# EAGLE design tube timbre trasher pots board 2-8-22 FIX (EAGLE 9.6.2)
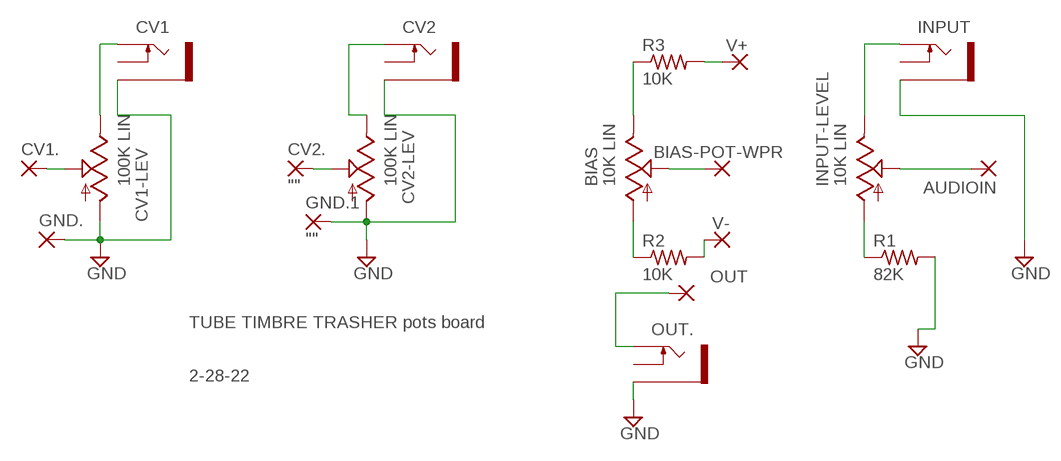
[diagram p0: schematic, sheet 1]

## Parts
AUDIOIN  WIREPAD3,17/1,3  [3,17/1,3]
BIAS  10K LIN  9MM_SNAP-IN_POT_  [9MM_SNAP-IN_POT]
BIAS-POT-WPR  WIREPAD3,17/1,3  [3,17/1,3]
CV1  THONKICONNNEW  [WQP-PJ301M-12_JACK]
CV1-LEV  100K LIN  9MM_SNAP-IN_POT_  [9MM_SNAP-IN_POT]
CV1.  WIREPAD3,17/1,3  [3,17/1,3]
CV2  THONKICONNNEW  [WQP-PJ301M-12_JACK]
CV2-LEV  100K LIN  9MM_SNAP-IN_POT_  [9MM_SNAP-IN_POT]
CV2.  ""  WIREPAD3,17/1,3  [3,17/1,3]
GND.  WIREPAD3,17/1,3  [3,17/1,3]
GND.1  ""  WIREPAD3,17/1,3  [3,17/1,3]
INPUT  THONKICONNNEW  [WQP-PJ301M-12_JACK]
INPUT-LEVEL  10K LIN  9MM_SNAP-IN_POT_  [9MM_SNAP-IN_POT]
OUT  WIREPAD3,17/1,3  [3,17/1,3]
OUT.  THONKICONNNEW  [WQP-PJ301M-12_JACK]
R1  82K  R-US_0207/10  [0207/10]
R2  10K  R-US_0207/10  [0207/10]
R3  10K  R-US_0207/10  [0207/10]
V+  WIREPAD3,17/1,3  [3,17/1,3]
V-  WIREPAD3,17/1,3  [3,17/1,3]

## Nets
GND: CV1-LEV.1(A) CV1.P$3_SLEEVE(SLEEVE) CV2-LEV.1(A) CV2.P$3_SLEEVE(SLEEVE) GND.1.1(P) GND..1(P) INPUT.P$3_SLEEVE(SLEEVE) OUT..P$3_SLEEVE(SLEEVE) R1.2
N$1: INPUT-LEVEL.3(E) INPUT.P$1_TIP(TIP)
N$2: AUDIOIN.1(P) INPUT-LEVEL.2(S)
N$3: BIAS.3(E) R3.1
N$4: OUT.1(P) OUT..P$1_TIP(TIP)
N$5: CV1-LEV.3(E) CV1.P$1_TIP(TIP)
N$6: CV2-LEV.3(E) CV2.P$1_TIP(TIP)
N$7: CV1-LEV.2(S) CV1..1(P)
N$8: CV2-LEV.2(S) CV2..1(P)
N$9: BIAS.1(A) R2.1
N$10: BIAS-POT-WPR.1(P) BIAS.2(S)
N$12: INPUT-LEVEL.1(A) R1.1
N$13: R3.2 V+.1(P)
N$14: R2.2 V-.1(P)
Unconnected: CV1.P$2_SWITCH(SWITCH) CV2.P$2_SWITCH(SWITCH) INPUT.P$2_SWITCH(SWITCH) OUT..P$2_SWITCH(SWITCH)

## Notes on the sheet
- TUBE TIMBRE TRASHER pots board
- 2-28-22

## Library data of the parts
AUDIOIN BIAS-POT-WPR CV1. CV2. GND. GND.1 OUT V+ V- = wirepad:WIREPAD: Wire PAD connect wire on PCB
BIAS CV1-LEV CV2-LEV INPUT-LEVEL = MusicThingModular:9MM_SNAP-IN_POT: 9mm vertical snap-in pot, Alpha / Panasonic style
CV1 CV2 INPUT OUT. = MusicThingModular-CL:THONKICONN: 3.5mm socket for Eurorack modular synths
R1-R3 = adafruit:R-US_: RESISTOR, American symbol

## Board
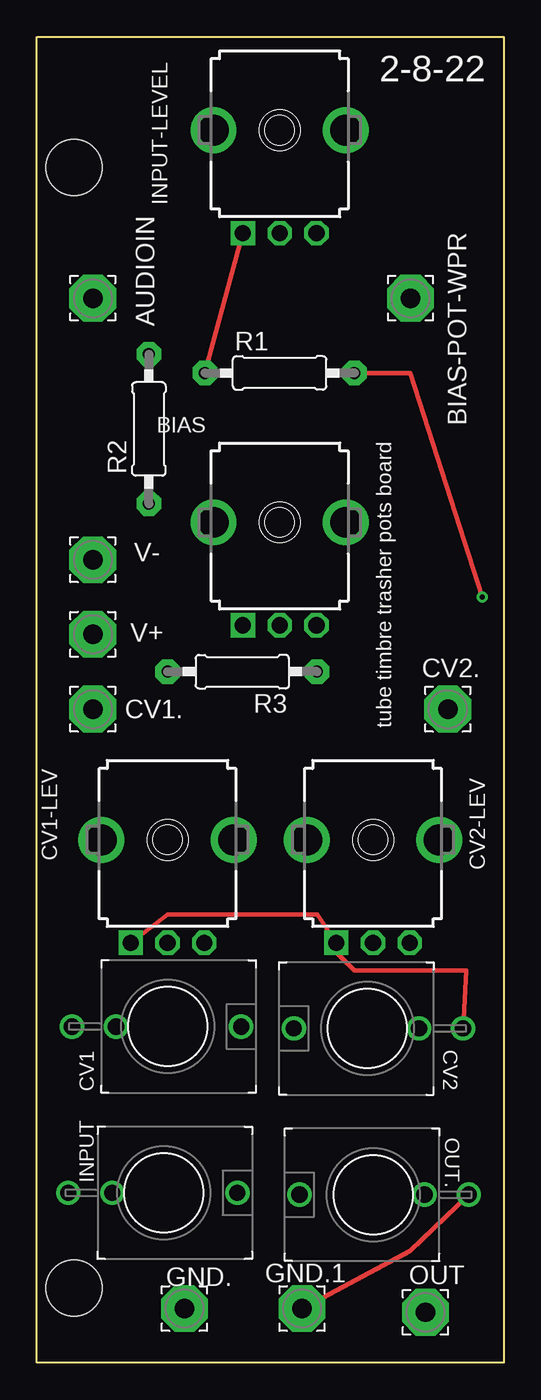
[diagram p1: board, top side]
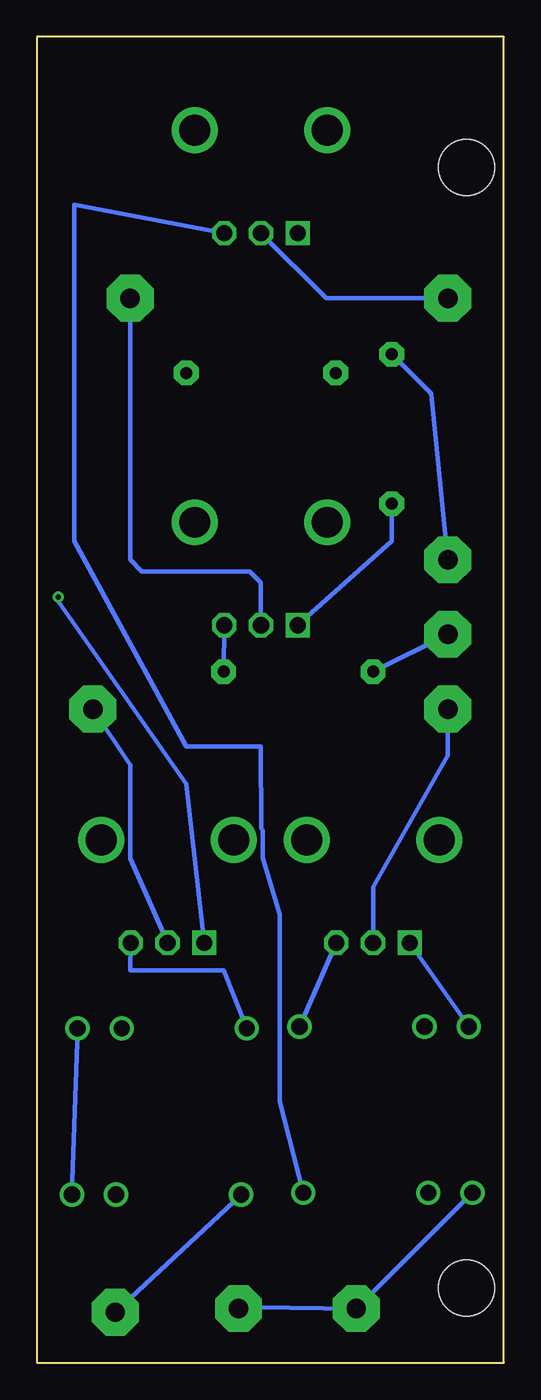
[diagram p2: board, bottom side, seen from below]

Size 31.75 x 90.17 mm. Coordinates in mm from the lower left corner, seen from the top.
Outline: 0,0 0,90.17 31.75,90.17 31.75,0 0,0
Copper layers (1*16): Top 0.035mm / dielectric 1.5mm / Bottom 0.035mm
Design rules "default": minimum track width 6mil, minimum drill 0.35mm, track to track 6mil, track to pad 6mil, pad to pad 6mil, via to via 6mil, smd to smd 6mil, copper to edge 40mil, drill to drill 6mil, minimum pad ring 10mil, minimum via ring 8mil, stop-mask expansion 4mil, vias tented up to drill 0mil, thermal gap 10mil
Holes 3.81 mm at 2.54,81.28 2.54,5.08

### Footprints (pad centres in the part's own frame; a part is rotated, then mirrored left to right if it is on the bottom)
3,17/1,3 = drill 1.321 pad 3.175 octagon: 1 0,0
9MM_SNAP-IN_POT = drill 1.1 square: 1 -2.5,-7 | drill 1.1 octagon: 2 0,-7; 3 2.5,-7 | drill 2.1 pad 2.794: CHASSIS1 -4.5,0; CHASSIS2 4.5,0
WQP-PJ301M-12_JACK = drill 1.1: P$1_TIP 0,5; P$2_SWITCH 0,-3.5; P$3_SLEEVE 0,-6.5
0207/10 = drill 0.813 pad 1.676 octagon: 1 -5.08,0; 2 5.08,0

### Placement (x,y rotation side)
AUDIOIN  3.81,72.39 0 top
BIAS  16.51,57.15 0 top
BIAS-POT-WPR  25.4,72.39 0 top
CV1  8.89,22.86 270 top
CV1-LEV  8.89,35.56 0 top
CV1.  3.81,44.45 0 top
CV2  22.48,22.73 90 top
CV2-LEV  22.86,35.56 0 top
CV2.  27.94,44.45 0 top
GND.  10.03,3.68 0 top
GND.1  18.03,3.68 0 top
INPUT  8.64,11.56 270 top
INPUT-LEVEL  16.51,83.82 0 top
OUT  26.42,3.43 0 top
OUT.  22.86,11.43 90 top
R1  16.51,67.31 0 top
R2  7.62,63.5 90 top
R3  13.97,46.99 180 top
V+  3.81,49.53 0 top
V-  3.81,54.61 0 top

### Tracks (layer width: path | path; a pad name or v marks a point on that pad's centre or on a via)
GND  (via drill 0.35)
  Top 0.305: GND.1.1 25.4,7.62 OUT..P$3_SLEEVE | v30.28,52.07 25.4,67.31 R1.2 | CV2.P$3_SLEEVE 29.21,26.67 21.59,26.67 20.36,27.9 CV2-LEV.1 19.05,30.48 8.89,30.48 CV1-LEV.1
  Bottom 0.305: GND.1.1 19.05,3.81 GND..1 2.16,11.56 INPUT.P$3_SLEEVE | CV1.P$3_SLEEVE CV1-LEV.1 | OUT..P$3_SLEEVE CV2.P$3_SLEEVE | CV2-LEV.1 21.59,39.37 30.48,52.07 v30.28,52.07
N$1
  Bottom 0.305: INPUT-LEVEL.3 29.21,78.74 29.21,55.88 21.59,41.91 16.51,41.91 16.5,36.33 16.38,36.21 16.38,34.33 15.24,30.48 15.24,17.78 INPUT.P$1_TIP
N$2
  Bottom 0.305: AUDIOIN.1 12.08,72.39 INPUT-LEVEL.2
N$3
  Bottom 0.305: R3.1 BIAS.3
N$4
  Bottom 0.305: OUT.1 OUT..P$1_TIP
N$5
  Bottom 0.305: CV1.P$1_TIP CV1-LEV.3
N$6
  Bottom 0.305: CV2.P$1_TIP 19.05,26.67 25.4,26.67 CV2-LEV.3
N$7
  Bottom 0.305: CV1-LEV.2 8.89,32.37 3.81,41.29 CV1..1
N$8
  Bottom 0.305: CV2-LEV.2 25.4,34.29 25.4,40.64 CV2..1
N$9
  Bottom 0.305: BIAS.1 7.62,55.88 R2.1
N$10
  Bottom 0.305: BIAS.2 16.51,53.06 17.27,53.82 24.61,53.82 25.4,54.61 BIAS-POT-WPR.1
N$12
  Top 0.305: R1.1 INPUT-LEVEL.1
N$13
  Bottom 0.305: R3.2 V+.1
N$14
  Bottom 0.305: V-.1 4.94,65.9 R2.2

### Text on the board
tNames: 2-8-22 | tube timbre trasher pots board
